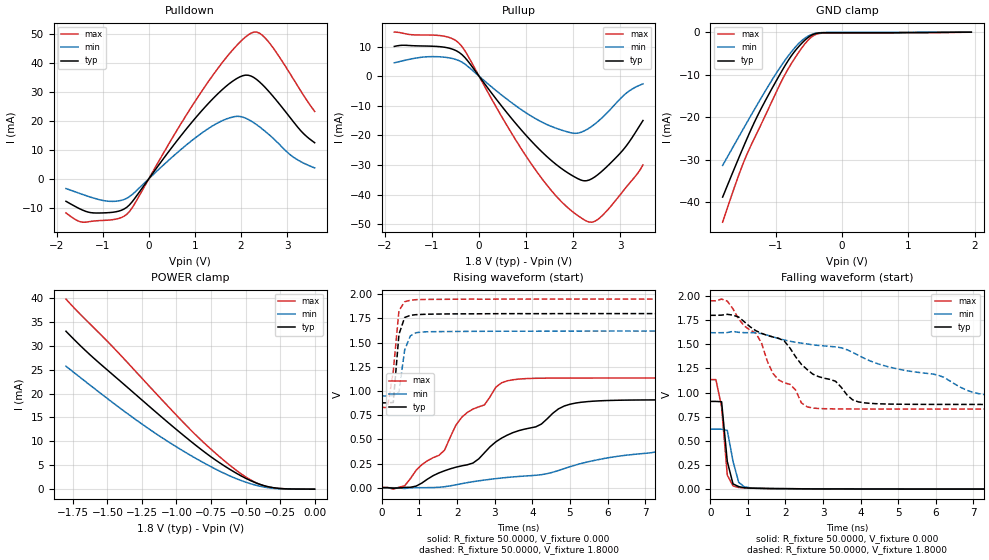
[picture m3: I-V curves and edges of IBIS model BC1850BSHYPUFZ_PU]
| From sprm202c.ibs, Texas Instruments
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|   Model BC1850BSHYPUFZ_PU
[Model]   BC1850BSHYPUFZ_PU
Model_type   I/O
Polarity   Non-Inverting
Enable   Active-Low
Vinl =   0.8500V
Vinh =   0.9800V
Vmeas =   0.9000V
Cref =  15.0000pF
Rref = 100.0000M
Vref =  0.000V
C_comp   1.2800pF   1.4600pF   1.1000pF
[Model Spec]
|   typ   min   max
Vinh   0.98V   0.86V   1.1V
Vinl   0.85V   0.70V   0.91V
[Temperature Range]   25.0000   0.1250k   -40.0000
[Voltage Range]   1.8000V   1.6200V   1.9500V
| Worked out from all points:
|   slope of the pulldown table from 0 to 0.27 V, typ, clamps not added: 45.4 ohm
|   slope of the pullup table from 0 to 0.27 V, typ, clamps not added: 46.7 ohm
|   GND clamp passes 1 mA (typ) near -0.49 V on its own axis
|   POWER clamp passes 1 mA (typ) near -0.40 V on its own axis
|   rising waveform, R_fixture 50.0000, V_fixture 0.000: 20-80 % time 2.71ns typ, 4.12ns min, 1.78ns max; typ from 0.003 V to 0.909 V
|   rising waveform, R_fixture 50.0000, V_fixture 1.8000: 20-80 % time 139ps typ, 183ps min, 186ps max; typ from 0.878 V to 1.8 V
|   falling waveform, R_fixture 50.0000, V_fixture 0.000: 20-80 % time 176ps typ, 213ps min, 163ps max; typ from 0.909 V to 0.003 V
|   falling waveform, R_fixture 50.0000, V_fixture 1.8000: 20-80 % time 2.11ns typ, 3.58ns min, 1.37ns max; typ from 1.8 V to 0.878 V
[Pulldown]
| voltage   I(typ)   I(min)   I(max)
-1.8V     -7.807mA   -3.392mA   -11.84mA
-1.44V    -10.87mA   -5.437mA   -15.06mA
-900mV    -11.77mA   -7.765mA   -14.36mA
-480mV    -9.903mA   -6.777mA   -12.32mA
720mV     15.38mA    10.45mA    19.67mA
1.38V     27.57mA    18.29mA    35.66mA
1.86V     34.25mA    21.54mA    45.36mA
2.22V     35.59mA    20mA       50.48mA
2.4V      33.61mA    18.03mA    50.47mA
2.58V     30.7mA     15.71mA    47.82mA
3.12V     20.13mA    7.698mA    35.04mA
3.6V      12.48mA    3.751mA    23.33mA
[Pullup]
| voltage   I(typ)   I(min)   I(max)
-1.8V     10.05mA    4.513mA    14.9mA
-1.08V    10.17mA    6.578mA    13.91mA
-660mV    9.558mA    6.262mA    13.21mA
-420mV    7.99mA     5.205mA    11.06mA
660mV     -13.69mA   -8.592mA   -18.48mA
1.2V      -23.44mA   -14.35mA   -31.69mA
1.92V     -33.02mA   -19.01mA   -44.92mA
2.28V     -35.33mA   -18.09mA   -48.94mA
2.46V     -33.99mA   -16.13mA   -49mA
2.64V     -31.65mA   -13.6mA    -46.71mA
3.12V     -23.67mA   -5.802mA   -37.58mA
3.48V     -14.97mA   -2.586mA   -30mA
[GND_clamp]
| voltage   I(typ)   I(min)   I(max)
-1.8V     -38.81mA   -31.35mA   -44.71mA
-1.6V     -31.22mA   -25.82mA   -35.51mA
-1.48V    -26.76mA   -22.52mA   -30.48mA
-1.28V    -19.86mA   -17.1mA    -23.65mA
-1.04V    -12.81mA   -10.86mA   -15.71mA
-880mV    -8.417mA   -7.07mA    -10.55mA
-720mV    -4.646mA   -3.807mA   -6.316mA
-560mV    -1.878mA   -1.411mA   -2.748mA
-440mV    -552.8uA   -426.4uA   -892.7uA
-360mV    -209.7uA   -154.5uA   -352.6uA
-280mV    -132uA     -75.21uA   -219uA
1.95V     14.01nA    25uA       0A
[POWER_clamp]
| voltage   I(typ)   I(min)   I(max)
-1.8V     33.03mA    25.71mA    39.76mA
-1.6V     27.43mA    21.18mA    33.81mA
-1.34V    20.91mA    15.49mA    26.02mA
-1.12V    15.39mA    11.06mA    19.14mA
-840mV    8.716mA    6.11mA     10.76mA
-720mV    6.145mA    4.242mA    7.585mA
-580mV    3.557mA    2.349mA    4.228mA
-500mV    2.291mA    1.48mA     2.583mA
-440mV    1.488mA    943.7uA    1.569mA
-340mV    539.6uA    314uA      490.5uA
-220mV    86.02uA    44.45uA    88.85uA
0V        13.12nA    71.97nA    15.04nA
[Ramp]
| variable   typ   min   max
dV/dt_r   0.5191/2.6576n   0.1340/2.5125n   0.6781/1.7821n
dV/dt_f   0.5517/2.1486n   0.2259/2.3696n   0.6717/1.4098n
R_load = 50.0000
[Rising Waveform]
R_fixture = 50.0000
V_fixture = 0.000
V_fixture_min = 0.000
V_fixture_max = 0.000
| time   V(typ)   V(min)   V(max)
0s        2.794mV    1.55mV     4.114mV
606.1ps   4.593mV    -6.614mV   21.06mV
1.061ns   49.19mV    2.42mV     238.8mV
1.667ns   176.7mV    11.93mV    389.8mV
1.97ns    213.6mV    31.71mV    648.5mV
2.424ns   256.8mV    64.06mV    814.6mV
3.333ns   544.6mV    107.8mV    1.106V
5.455ns   890.3mV    266.8mV    1.135V
9.091ns   909.2mV    584.2mV    1.135V
15ns      909.3mV    621.9mV    1.135V
[Rising Waveform]
R_fixture = 50.0000
V_fixture = 1.8000
V_fixture_min = 1.6200
V_fixture_max = 1.9500
| time   V(typ)   V(min)   V(max)
0s        877.9mV    949.5mV    830.5mV
151.5ps   878.1mV    949.5mV    830.6mV
303ps     882mV      950mV      1.202V
454.5ps   1.585V     990.2mV    1.831V
606.1ps   1.76V      1.423V     1.922V
757.6ps   1.782V     1.57V      1.938V
909.1ps   1.789V     1.603V     1.944V
1.061ns   1.792V     1.609V     1.945V
1.515ns   1.795V     1.614V     1.947V
15ns      1.8V       1.62V      1.95V
[Falling Waveform]
R_fixture = 50.0000
V_fixture = 0.000
V_fixture_min = 0.000
V_fixture_max = 0.000
| time   V(typ)   V(min)   V(max)
0s        909.3mV    622.2mV    1.135V
151.5ps   909.3mV    622.2mV    1.135V
303ps     906.2mV    622.2mV    853.9mV
454.5ps   287.5mV    609.6mV    147.1mV
606.1ps   56.49mV    291.1mV    35.68mV
757.6ps   28.14mV    71.97mV    18.6mV
909.1ps   16.4mV     26.18mV    14.08mV
1.061ns   12.3mV     16.3mV     12.04mV
1.818ns   7.793mV    6.519mV    6.577mV
15ns      2.797mV    1.683mV    4.114mV
[Falling Waveform]
R_fixture = 50.0000
V_fixture = 1.8000
V_fixture_min = 1.6200
V_fixture_max = 1.9500
| time   V(typ)   V(min)   V(max)
0s        1.8V       1.62V      1.95V
454.5ps   1.81V      1.622V     1.947V
1.212ns   1.641V     1.619V     1.616V
1.667ns   1.576V     1.578V     1.2V
1.97ns    1.534V     1.545V     1.101V
2.727ns   1.192V     1.494V     841.1mV
3.333ns   1.118V     1.473V     832mV
3.939ns   904.5mV    1.386V     830.9mV
7.424ns   878mV      972.8mV    830.5mV
15ns      877.9mV    950.9mV    830.5mV
